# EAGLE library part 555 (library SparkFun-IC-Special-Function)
General purpose bipolar Timer Datasheet SparkFun Products SparkFun SparkPunk Sequencer Kit (KIT-12707) Storefront Component: 555 Timer (COM-09273) Two parts valid for production: VFP: IC-11930 (M7555 PTH) VFP: IC-09173 (555 PTH) - Preferred
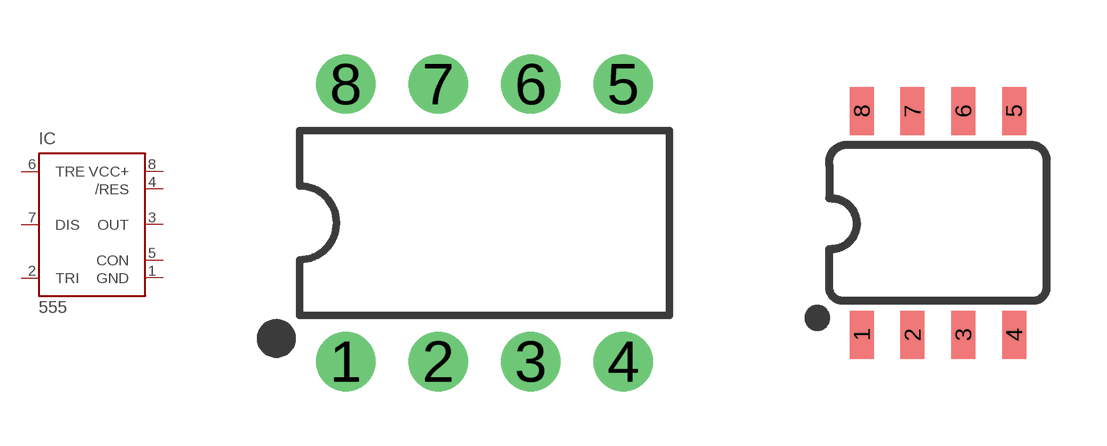
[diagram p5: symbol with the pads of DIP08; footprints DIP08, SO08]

Designator prefix IC

## 555P (PROD_ID: IC-09173; PROD_ID_ALT: IC-09173; VALUE: 555)  [DIP08]
1  GND  pwr
2  TRI  in
3  OUT  out
4  /RES  in
5  CON  in
6  TRE  in
7  DIS  in
8  VCC+  pwr

## 555D (PROD_ID: NA-XXXXX; VALUE: 555)  [SO08]
Pads as for DIP08

## 555KIT (PROD_ID: IC-09173; PROD_ID_ALT: IC-11930; VALUE: 555)  [DIP08-KIT]
Pads as for DIP08

## Footprint DIP08 (pad centres in mm)
Dual In Line Package
drill 0.813 pad 1.626: 1 -3.81,-3.81; 2 -1.27,-3.81; 3 1.27,-3.81; 4 3.81,-3.81; 5 3.81,3.81; 6 1.27,3.81; 7 -1.27,3.81; 8 -3.81,3.81

## Footprint SO08 (pad centres in mm)
SOIC, 0.15 inch width
smd 0.6 x 1.2: 1 -1.905,-2.8; 2 -0.635,-2.8; 3 0.635,-2.8; 4 1.905,-2.8; 5 1.905,2.8; 6 0.635,2.8; 7 -0.635,2.8; 8 -1.905,2.8

## Footprint DIP08-KIT (pad centres in mm)
drill 0.813 pad 1.905: 1 -3.81,-4.191; 2 -1.27,-4.191; 3 1.27,-4.191; 4 3.81,-4.191; 5 3.81,4.191; 6 1.27,4.191; 7 -1.27,4.191
drill 0.864 pad 1.905: 8 -3.81,4.191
